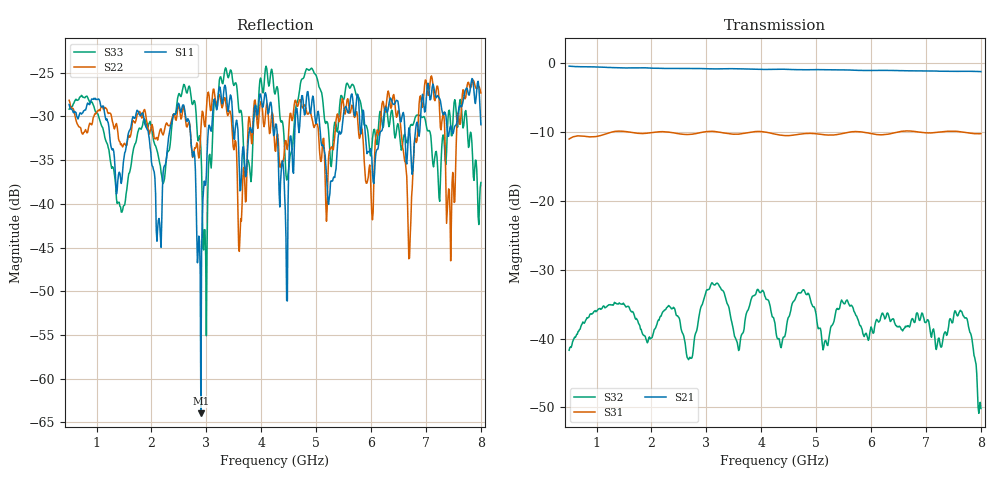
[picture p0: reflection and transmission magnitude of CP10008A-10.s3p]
! Amtery
! Email: info@amtery.com
! Phone: 886-2-2883-7839
! Model Number: CP10008-10
! 3-port S-parameter measurement data for Directional Coupler
! Frequency Range: 0.5 GHz to 8 GHz
! Port 1: Input
! Port 2: Output
! Port 3: Coupled
# Hz S ma R 50
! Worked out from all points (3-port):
!   601 points, 500 MHz to 8 GHz, reference 50 ohm
!   strongest paths, dB at 500 MHz, 2.375 GHz, 4.25 GHz, 6.125 GHz, 8 GHz:
!     S21: -0.5, -0.8, -0.9, -1.1, -1.3
!     S31: -11.1, -10.1, -10.3, -10.4, -10.3
!     S32: -41.7, -35.7, -37.8, -37.5, -50.1
!   lowest |S11| = -64.0 dB at 2.9 GHz (marker M1), VSWR 1.00, Z = 50 + j0.0516 ohm
!   |S11| at or under -10 dB: start of sweep to end of sweep
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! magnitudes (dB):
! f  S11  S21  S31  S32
! 500 MHz  -28.6  -0.5  -11.1  -41.7
! 2.138 GHz  -41.7  -0.8  -10.0  -37.3
! 2.587 GHz  -28.7  -0.8  -10.4  -39.6
! 2.9 GHz  -64.0  -0.8  -10.1  -35.5
! 3.237 GHz  -26.6  -0.9  -10.1  -32.4
! 3.612 GHz  -38.5  -0.9  -10.3  -40.7
! 4.25 GHz  -31.4  -0.9  -10.3  -37.8
! 6.7 GHz  -31.5  -1.2  -9.9  -38.3
! 7.612 GHz  -28.8  -1.2  -10.0  -36.1
! 8 GHz  -30.9  -1.3  -10.3  -50.1
